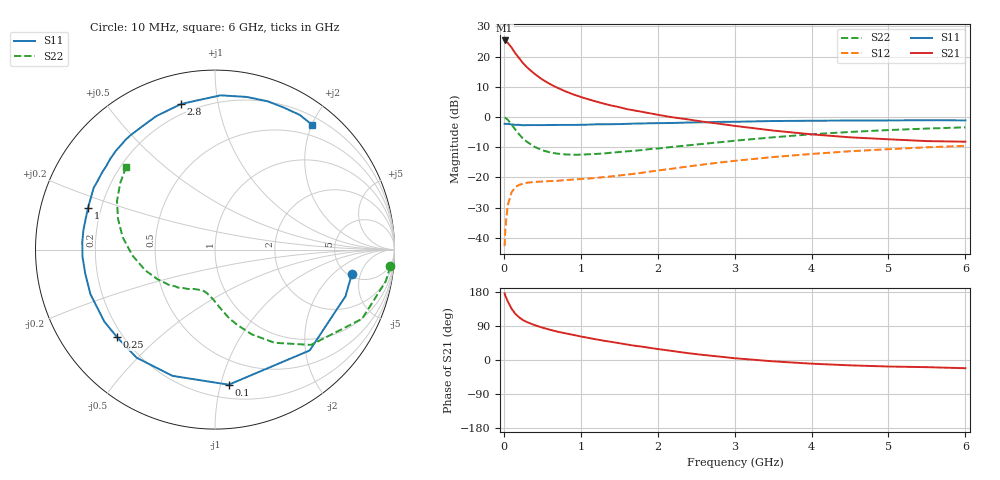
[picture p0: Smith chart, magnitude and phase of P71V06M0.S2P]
! SIEMENS Small Signal Semiconductors
! BFP196
! Si NPN RF Bipolar Junction Transistor in SOT143
! VCE = 1 V  IC = 6 mA
! Common Emitter S-Parameters:  May  1996
# GHz  S  MA  R  50
!  f  S11  S21  S12  S22
! GHz  MAG  ANG  MAG  ANG  MAG  ANG  MAG  ANG
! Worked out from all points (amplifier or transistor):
!   36 points, 10 MHz to 6 GHz, reference 50 ohm
!   highest |S21| = 25.4 dB at 10 MHz (marker M1)
!   |S21| within 3 dB of that: start of sweep to 117.3 MHz
!   unconditionally stable (mu >= 1): 1.015 GHz to end of sweep
!   at 250 MHz: K = 0.30, MSG = 20.0 dB, |S12| = -22.1 dB
!   at 1.4 GHz: K = 1.18, MAG = 9.2 dB, |S12| = -19.6 dB
!   at 6 GHz: K = 1.04, MAG = -0.5 dB, |S12| = -9.5 dB
!   S11 on the Smith chart (normalised r, x): 10 MHz: 5.31, -3.63; 100 MHz: 0.30, -1.06; 250 MHz: 0.18, -0.37; 1 GHz: 0.15, +0.16; 2.8 GHz: 0.15, +0.78; 6 GHz: 0.32, +2.00
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0.01  0.7742 -10.2  18.52 175.7  0.0073 86.1  0.9812 -5.5
0.02  0.7721 -19.7  17.99 169.4  0.0146 80.2  0.9678 -10.5
0.05  0.7707 -46.8  16.95 155.0  0.0344 66.9  0.9058 -25.2
0.1  0.7566 -84.2  14.16 135.5  0.0568 50.4  0.7536 -44.8
0.15  0.7423 -108.6  11.33 121.7  0.0692 40.2  0.6164 -57.4
0.2  0.7439 -126.0  9.388 112.3  0.0756 33.4  0.5152 -66.5
0.25  0.732 -138.4  7.804 105.2  0.0789 28.9  0.4387 -73.4
0.3  0.7356 -147.0  6.675 100.1  0.0818 26.6  0.3899 -78.4
0.4  0.7372 -160.4  5.178 92.1  0.0845 23.5  0.3216 -85.6
0.5  0.7353 -169.5  4.19 85.5  0.0857 22.2  0.2822 -91.3
0.6  0.7396 -177.1  3.519 79.8  0.0872 21.9  0.2602 -96.1
0.7  0.7405 176.6  3.039 74.7  0.0883 22.6  0.2477 -100.1
0.8  0.7412 171.6  2.665 70.4  0.0906 23.2  0.241 -103.8
1  0.7449 161.7  2.151 62.1  0.0942 25.1  0.2388 -109.5
1.1  0.7494 157.4  1.966 58.2  0.0961 26.6  0.2421 -112.8
1.6  0.7723 139.0  1.353 40.9  0.1115 32.4  0.2708 -126.6
2.2  0.7984 119.9  0.988 23.5  0.1404 35.7  0.3218 -141.8
2.8  0.8325 103.2  0.775 9.1  0.1765 34.1  0.3824 -158.7
3.5  0.8601 87.9  0.598 -3.5  0.2179 28.0  0.462 -176.1
4.5  0.877 70.4  0.462 -14.1  0.2716 17.1  0.5671 162.4
5.5  0.8866 57.8  0.4 -18.9  0.3157 5.5  0.645 145.0
6  0.8809 52.2  0.391 -21.7  0.3348 -0.9  0.6758 137.2
